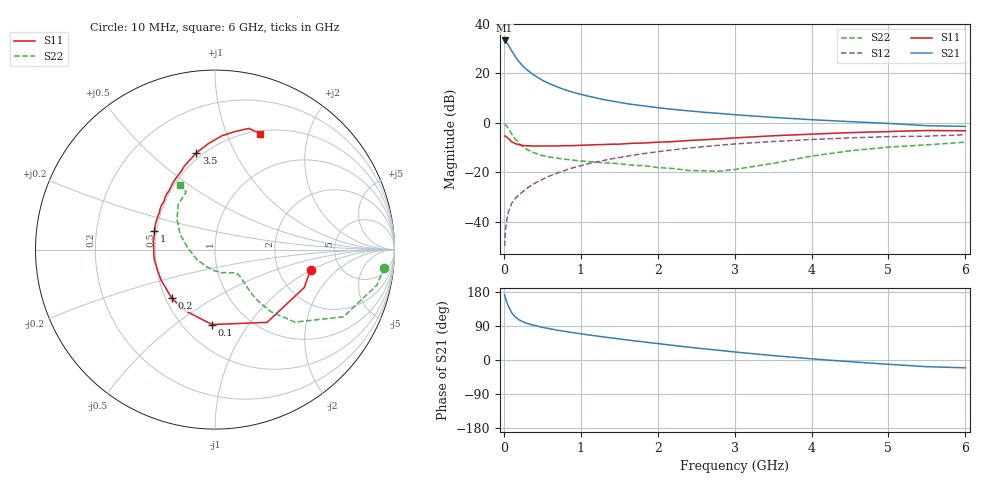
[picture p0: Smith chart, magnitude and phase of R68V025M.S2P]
! SIEMENS Small Signal Semiconductors
! BFR193
! Si NPN RF Bipolar Junction Transistor in SOT23
! VCE = 8 V  IC = 25 mA
! Common Emitter S-Parameters:  May  1996
# GHz  S  MA  R  50
!  f  S11  S21  S12  S22
! GHz  MAG  ANG  MAG  ANG  MAG  ANG  MAG  ANG
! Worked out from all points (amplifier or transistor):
!   36 points, 10 MHz to 6 GHz, reference 50 ohm
!   highest |S21| = 33.4 dB at 10 MHz (marker M1)
!   |S21| within 3 dB of that: start of sweep to 79.63 MHz
!   unconditionally stable (mu >= 1): 566.2 MHz to 2.121 GHz
!   at 250 MHz: K = 0.86, MSG = 25.3 dB, |S12| = -27.7 dB
!   at 1.4 GHz: K = 1.02, MAG = 10.8 dB, |S12| = -14.6 dB
!   at 6 GHz: K = 0.94, MSG = 1.7 dB, |S12| = -4.8 dB
!   S11 on the Smith chart (normalised r, x): 10 MHz: 3.05, -0.96; 100 MHz: 0.68, -0.69; 200 MHz: 0.54, -0.34; 1 GHz: 0.49, +0.11; 3.5 GHz: 0.46, +0.71; 6 GHz: 0.53, +1.32
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0.01  0.5438 -11.8  46.63 171.9  0.0032 84.8  0.9494 -6.1
0.02  0.5405 -23.0  45.24 164.5  0.0066 79.1  0.9238 -12.3
0.05  0.4985 -54.4  39.71 145.8  0.0142 70.3  0.8082 -27.6
0.1  0.4178 -92.3  29.08 125.3  0.0234 65.0  0.6013 -42.2
0.15  0.3787 -116.2  21.73 113.2  0.0297 63.6  0.4661 -48.0
0.2  0.3627 -131.6  17.18 105.8  0.0353 64.3  0.3815 -49.9
0.25  0.3478 -142.2  14.03 100.6  0.0411 65.7  0.3259 -50.3
0.3  0.3452 -150.9  11.87 96.8  0.0472 67.1  0.2914 -49.9
0.4  0.3401 -162.5  9.093 91.2  0.0598 68.8  0.2465 -48.6
0.5  0.3424 -171.0  7.312 86.3  0.0718 69.7  0.2181 -47.4
0.6  0.3419 -176.8  6.151 82.3  0.085 69.8  0.2028 -46.9
0.7  0.3423 176.8  5.305 78.5  0.0975 69.3  0.1925 -47.1
0.8  0.3465 171.7  4.66 75.3  0.1103 68.6  0.1833 -47.4
1  0.3524 163.1  3.786 69.2  0.1361 67.4  0.1701 -49.2
1.1  0.3566 159.5  3.468 66.3  0.1491 66.5  0.1655 -51.7
1.6  0.3815 143.1  2.451 53.0  0.2118 60.5  0.1433 -64.3
2.2  0.4181 127.4  1.877 38.6  0.2852 52.5  0.1193 -89.7
2.8  0.4751 113.4  1.556 25.5  0.3537 43.7  0.1052 -134.0
3.5  0.5487 101.0  1.293 11.6  0.4204 33.0  0.1517 176.6
4.5  0.6357 86.5  1.061 -4.5  0.4986 19.0  0.2725 141.1
5.5  0.7011 74.4  0.878 -17.7  0.5402 5.1  0.3598 116.5
6  0.6935 68.7  0.85 -20.6  0.5759 1.1  0.4079 118.2
